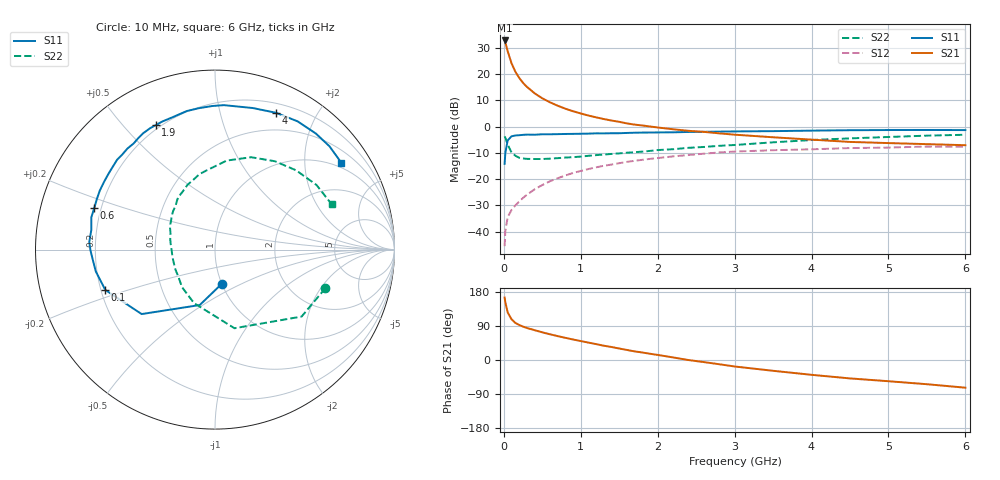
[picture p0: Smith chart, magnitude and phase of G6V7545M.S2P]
! SIEMENS Small Signal Semiconductors
! BFG193
! Si NPN RF Bipolar Junction Transistor in SOT223
! VCE = 0.75 V  IC = 45 mA
! Common Emitter S-Parameters:  August  1996
# GHz  S  MA  R  50
!  f  S11  S21  S12  S22
! GHz  MAG  ANG  MAG  ANG  MAG  ANG  MAG  ANG
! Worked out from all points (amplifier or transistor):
!   36 points, 10 MHz to 6 GHz, reference 50 ohm
!   highest |S21| = 32.7 dB at 10 MHz (marker M1)
!   |S21| within 3 dB of that: start of sweep to 39.93 MHz
!   unconditionally stable (mu >= 1): start of sweep to 12.84 MHz; 199.8 MHz to end of sweep
!   at 250 MHz: K = 1.06, MAG = 20.4 dB, |S12| = -27.2 dB
!   at 1.4 GHz: K = 1.16, MAG = 5.9 dB, |S12| = -14.5 dB
!   at 6 GHz: K = 1.06, MAG = -1.1 dB, |S12| = -7.7 dB
!   S11 on the Smith chart (normalised r, x): 10 MHz: 1.00, -0.40; 100 MHz: 0.22, -0.17; 600 MHz: 0.17, +0.16; 1.9 GHz: 0.18, +0.62; 4 GHz: 0.30, +1.50; 6 GHz: 0.84, +3.00
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0.01  0.1948 -79.0  43.3 164.7  0.0053 75.7  0.6514 -19.3
0.02  0.3204 -105.4  39.48 151.8  0.0105 66.9  0.6099 -37.7
0.05  0.5442 -138.7  26.98 125.5  0.0189 54.1  0.4514 -76.1
0.1  0.6512 -159.8  15.95 107.4  0.0259 52.1  0.3202 -111.4
0.15  0.675 -169.6  11 97.9  0.0316 54.2  0.2784 -131.4
0.2  0.683 -175.1  8.416 92.4  0.0376 57.4  0.2542 -143.1
0.25  0.694 -179.7  6.747 88.1  0.0439 59.6  0.2469 -153.4
0.3  0.7017 176.6  5.673 84.5  0.0504 60.6  0.2424 -159.4
0.4  0.6977 171.0  4.284 78.7  0.0639 61.7  0.2408 -170.1
0.5  0.7121 165.4  3.435 73.0  0.0771 61.3  0.241 -177.9
0.6  0.7114 161.1  2.884 67.9  0.0909 60.3  0.2448 176.7
0.8  0.7211 152.9  2.181 58.5  0.1172 56.9  0.2566 166.6
1.1  0.7325 141.4  1.615 45.9  0.1553 50.8  0.2773 154.5
1.5  0.7451 127.5  1.227 30.3  0.2005 41.0  0.3082 141.0
1.9  0.7683 115.4  1.001 16.5  0.2423 31.3  0.3434 128.3
2.2  0.7753 107.1  0.887 6.8  0.2704 23.4  0.3698 119.2
2.8  0.8 91.2  0.741 -11.2  0.3211 8.4  0.4293 101.7
3.5  0.8163 75.1  0.624 -28.5  0.3541 -9.7  0.5003 82.5
4  0.8348 65.9  0.563 -39.1  0.3683 -19.3  0.5528 68.6
4.5  0.8499 57.2  0.509 -48.6  0.3891 -28.9  0.595 55.8
5.5  0.8592 42.1  0.462 -63.9  0.4159 -50.8  0.6704 32.5
6  0.8543 34.6  0.441 -73.1  0.412 -63.2  0.6969 21.3
